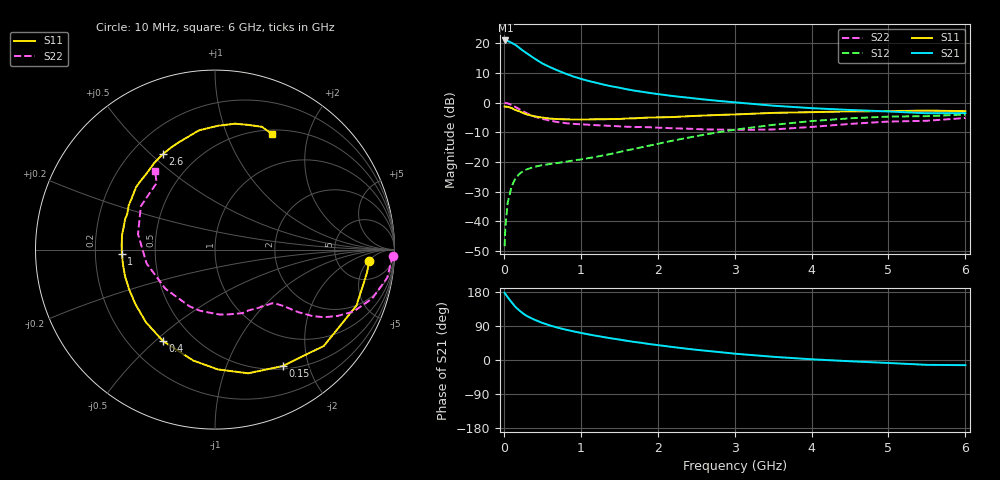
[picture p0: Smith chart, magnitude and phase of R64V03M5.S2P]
! SIEMENS Small Signal Semiconductors
! BFR193
! Si NPN RF Bipolar Junction Transistor in SOT23
! VCE = 4 V  IC = 3.5 mA
! Common Emitter S-Parameters:  May  1996
# GHz  S  MA  R  50
!  f  S11  S21  S12  S22
! GHz  MAG  ANG  MAG  ANG  MAG  ANG  MAG  ANG
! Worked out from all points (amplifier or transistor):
!   36 points, 10 MHz to 6 GHz, reference 50 ohm
!   highest |S21| = 20.9 dB at 20 MHz (marker M1)
!   |S21| within 3 dB of that: start of sweep to 226.7 MHz
!   unconditionally stable (mu >= 1): 999.9 MHz to 1.998 GHz
!   at 250 MHz: K = 0.33, MSG = 20.3 dB, |S12| = -23.1 dB
!   at 1.4 GHz: K = 1.09, MAG = 9.6 dB, |S12| = -17.3 dB
!   at 6 GHz: K = 0.98, MSG = 0.2 dB, |S12| = -4.0 dB
!   S11 on the Smith chart (normalised r, x): 10 MHz: 11, -5; 150 MHz: 0.54, -1.61; 400 MHz: 0.34, -0.53; 1 GHz: 0.32, -0.02; 2.6 GHz: 0.32, +0.54; 6 GHz: 0.55, +1.47
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0.01  0.8613 -4.3  10.99 177.4  0.0038 87.8  0.9938 -1.9
0.02  0.8565 -8.7  11.15 174.1  0.008 83.1  0.9838 -3.8
0.05  0.8478 -21.6  10.96 165.7  0.0205 77.7  0.9722 -9.3
0.1  0.8098 -41.5  10.21 152.7  0.0384 69.3  0.9171 -17.3
0.15  0.7505 -59.8  9.395 140.2  0.0524 60.5  0.8454 -24.1
0.2  0.7135 -75.0  8.397 131.0  0.0625 55.0  0.7769 -28.4
0.25  0.6678 -88.6  7.484 122.8  0.07 49.8  0.715 -31.8
0.3  0.6302 -101.0  6.759 116.0  0.0751 47.1  0.6596 -34.2
0.4  0.5867 -119.4  5.518 106.2  0.0828 43.4  0.5808 -36.9
0.5  0.5587 -133.4  4.571 98.0  0.0882 41.8  0.5314 -38.3
0.6  0.5378 -145.4  3.957 91.1  0.0921 41.8  0.4962 -39.4
0.7  0.5273 -155.3  3.477 85.3  0.0961 43.3  0.4697 -40.7
0.8  0.5226 -163.5  3.087 80.3  0.1004 44.4  0.4506 -41.8
1  0.5194 -177.3  2.517 71.6  0.11 47.9  0.4309 -44.7
1.1  0.5204 176.9  2.32 67.6  0.1159 49.8  0.4236 -46.8
1.6  0.5405 152.8  1.675 50.6  0.1564 57.7  0.3919 -58.5
2.2  0.5706 131.7  1.288 34.1  0.229 59.4  0.3692 -77.7
2.6  0.6055 118.8  1.13 24.9  0.2871 56.4  0.3531 -94.3
3.5  0.6706 97.6  0.887 8.5  0.4214 43.1  0.3522 -141.8
4.5  0.7102 81.0  0.751 -3.3  0.5436 24.9  0.4374 168.7
5.5  0.7324 69.1  0.661 -12.8  0.5913 6.8  0.4936 131.2
6  0.7181 63.6  0.665 -13.6  0.6281 1.7  0.5501 127.4
